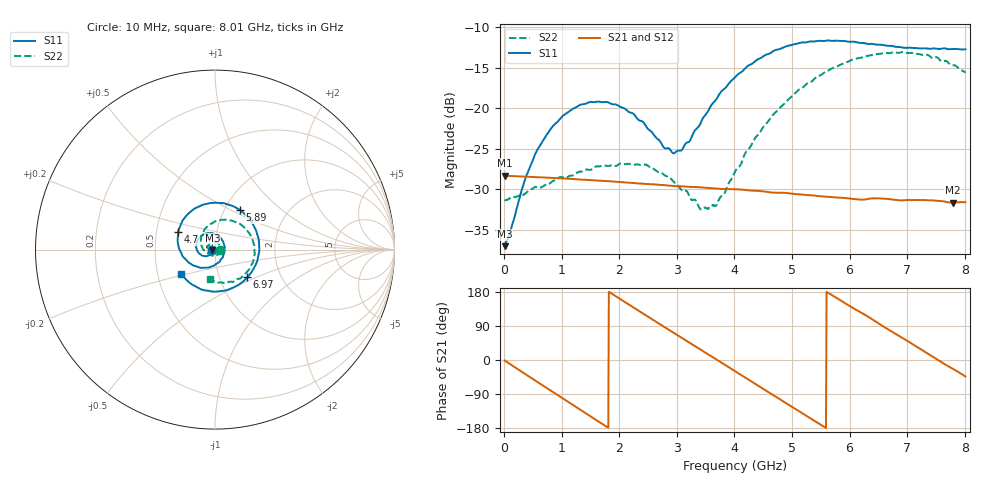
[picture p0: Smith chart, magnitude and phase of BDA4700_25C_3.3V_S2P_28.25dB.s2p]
!Agilent Technologies,E5071B,MY42404982,A.09.10
!Date: Mon Oct 20 18:14:57 2025
!Data & Calibration Information:
!Freq	S11:SOLT2(ON)	S21:SOLT2(ON)	S12:SOLT2(ON)	S22:SOLT2(ON)
# Hz S RI R 50
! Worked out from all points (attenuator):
!   801 points, 10 MHz to 8.01 GHz, reference 50 ohm
!   highest |S21| = -28.29 dB at 10 MHz (marker M1); lowest = -31.7 dB at 7.79 GHz (marker M2)
!   lowest |S11| = -37.0 dB at 10 MHz (marker M3), VSWR 1.03, Z = 48.6 - j0.127 ohm
!   |S11| at or under -10 dB: start of sweep to end of sweep
!   |S22| runs from -32.5 to -13.0 dB; largest |S21 - S12| = 0.00049
!   S11 on the Smith chart (normalised r, x): 10 MHz: 0.97, -0.00; 4.7 GHz: 0.65, +0.14; 5.89 GHz: 1.18, +0.56; 6.97 GHz: 1.35, -0.44; 8.01 GHz: 0.66, -0.19
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1e7  -0.014 -0.0013  0.0385 -0.000824  0.0384 -0.000861  0.0271 -0.000802
3.6e8  -0.0248 -0.0261  0.0305 -0.0224  0.0305 -0.0224  0.0227 -0.019
5.8e8  -0.0423 -0.0362  0.0199 -0.0319  0.0199 -0.0319  0.0145 -0.0292
1e9  -0.0849 -0.0242  -0.00616 -0.0364  -0.00617 -0.0365  -0.0146 -0.0348
1.35e9  -0.105 0.0142  -0.0252 -0.0261  -0.0252 -0.0262  -0.0364 -0.0183
1.97e9  -0.0585 0.0869  -0.034 0.00884  -0.0341 0.00882  -0.0348 0.0277
2.46e9  0.0181 0.0761  -0.0161 0.0301  -0.0161 0.0301  -0.00303 0.0447
2.68e9  0.0444 0.0465  -0.00415 0.0335  -0.00421 0.0335  0.0127 0.0383
2.93e9  0.0529 0.00175  0.00961 0.0318  0.00958 0.0317  0.025 0.0256
3.06e9  0.0496 -0.0232  0.0161 0.0288  0.0158 0.029  0.0279 0.0157
3.44e9  9.46e-05 -0.085  0.0295 0.0136  0.0296 0.0136  0.0198 -0.0136
3.69e9  -0.0546 -0.1006  0.032 0.000576  0.032 0.000501  0.00164 -0.0252
4.01e9  -0.1329 -0.0808  0.0276 -0.0155  0.0276 -0.0155  -0.031 -0.0259
4.7e9  -0.2058 0.0996  -0.00269 -0.03  -0.00254 -0.0301  -0.0795 0.0496
5.35e9  -0.0553 0.2529  -0.0267 -0.0114  -0.0266 -0.0116  -0.0159 0.1467
5.89e9  0.1393 0.2205  -0.0249 0.0128  -0.0249 0.0127  0.104 0.1577
6.28e9  0.2298 0.1032  -0.013 0.0241  -0.0126 0.0242  0.1842 0.0998
6.68e9  0.2373 -0.0543  0.00494 0.0271  0.00503 0.0271  0.2198 0.000468
6.97e9  0.1792 -0.1546  0.0161 0.0218  0.0162 0.0217  0.208 -0.0764
7.41e9  0.0216 -0.2324  0.0265 0.00556  0.0265 0.00555  0.1271 -0.1635
7.79e9  -0.1271 -0.1949  0.024 -0.0103  0.024 -0.0103  0.0231 -0.1835
8.01e9  -0.1889 -0.1345  0.0192 -0.0182  0.0193 -0.0181  -0.0297 -0.1637
